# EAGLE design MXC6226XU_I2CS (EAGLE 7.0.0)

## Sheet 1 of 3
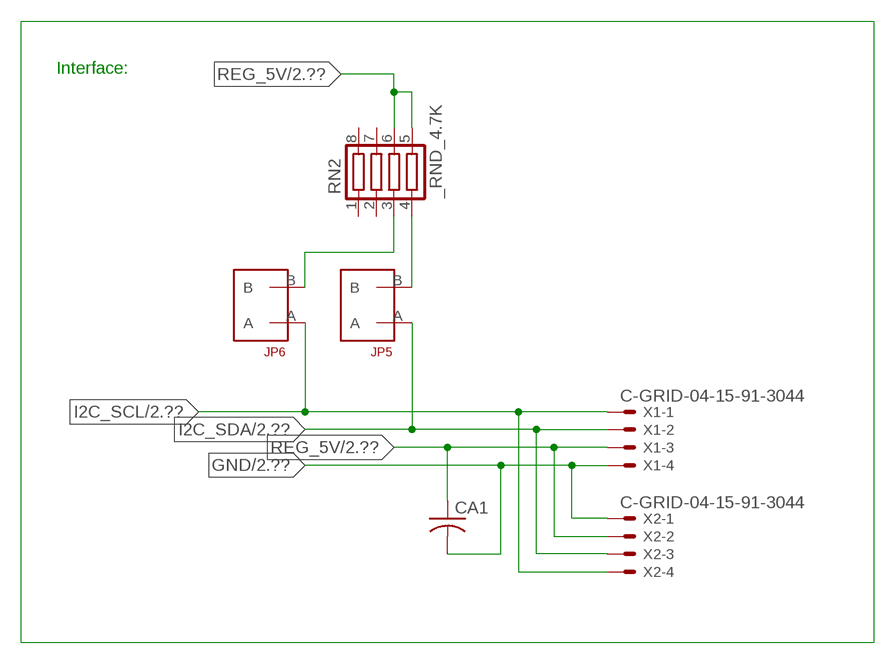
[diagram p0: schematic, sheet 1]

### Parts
CA1  CC1206KRX7R9BB104  [.1UF]
JP5  JUMPER_1X2_2MM  [JUMPER_1X2_2MM]
JP6  JUMPER_1X2_2MM  [JUMPER_1X2_2MM]
RN2  _RND_4.7K  [RND]
X1  C-GRID-04-15-91-3044  [15-91-04]
X2  C-GRID-04-15-91-3044  [15-91-04]

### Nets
GND: CA1.2 X1.4 X2.1 ; also sheet 2,3
I2C_SCL: JP6.A X1.1 X2.4 ; also sheet 2
I2C_SDA: JP5.A X1.2 X2.3 ; also sheet 2
N$1: JP6.B RN2.3
N$2: JP5.B RN2.4
REG_5V: CA1.1 RN2.5 RN2.6 X1.3 X2.2 ; also sheet 2,3
Unconnected: RN2.1 RN2.2 RN2.7 RN2.8

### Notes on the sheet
- Interface:

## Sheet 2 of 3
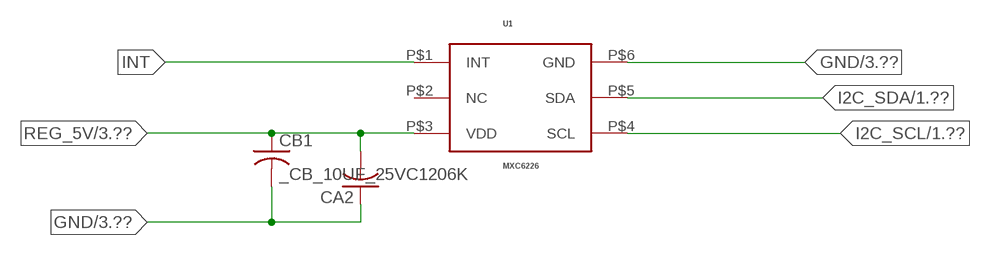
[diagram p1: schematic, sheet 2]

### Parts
CA2  _CA_.10UF_50VC1206K  [_CA_.1UF_50V]
CB1  _CB_10UF_25VC1206K  [_CB_10UF_25V]
U1  MXC6226  [MXC6226]

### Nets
GND: CA2.1 CB1.2 U1.P$6(GND) ; also sheet 1,3
I2C_SCL: U1.P$4(SCL) ; also sheet 1
I2C_SDA: U1.P$5(SDA) ; also sheet 1
INT: U1.P$1(INT)
REG_5V: CA2.2 CB1.1 U1.P$3(VDD) ; also sheet 1,3
Unconnected: U1.P$2(NC)

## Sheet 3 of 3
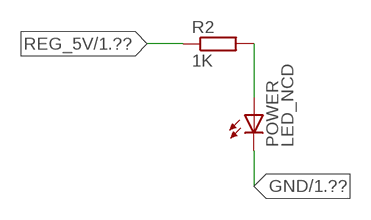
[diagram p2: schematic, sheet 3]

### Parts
POWER  LED_NCD  [CHIPLED_0603]
R2  1K  RESISTOR_SMT-0402  [R402]

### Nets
GND: POWER.C ; also sheet 1,2
N$3: POWER.A R2.2
REG_5V: R2.1 ; also sheet 1,2

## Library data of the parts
CA1 = NCD_ULTIMATE_LIBRARY:CC1206KRX7R9BB104: Capacitor CA .1uF 50V SMT C1206K CC1206KRX7R9BB104
CA2 = NCD_ULTIMATE_LIBRARY:_CA_.10UF_50V: Capacitor .1uF SMT
CB1 = NCD_ULTIMATE_LIBRARY:_CB_10UF_25V: Capacitor 10uF SMT
JP5 JP6 = NCD_ULTIMATE_CONNECTORS:JUMPER_1X2_2MM
POWER = NCD_ULTIMATE_LIBRARY:LED_NCD: LED Digikey 754-1132-2-ND/APT2012SRCPRV
R2 = NCD_ULTIMATE_LIBRARY:RESISTOR_SMT: NCD Resistor
RN2 = NCD_ULTIMATE_LIBRARY:_RND_4.7K: Resistor Array RND SMT 4.7K x 4 Single Resistor Source: http://www.ctscorp.com/components/Datasheets/CTSChipArrayDs.pdf Digikey 742C083472JPTR-ND/742C083472JP; OC_FARNELL: unknown; OC_NEWARK: unknown
U1 = NCD_ULTIMATE_bhaskar:MXC6226: http://www.memsic.com/userfiles/files/Datasheets/Accelerometer-Datasheets/MXC6226XU_Rev_1_3.pdf
X1 X2 = NCD_ULTIMATE_CONNECTORS:C-GRID-04: CONNECTOR 4-Pos I2C wire to board 2.54 mm (0.100") pitch header Digikey WM1342-ND/0015912045; OC_FARNELL: unknown; OC_NEWARK: unknown

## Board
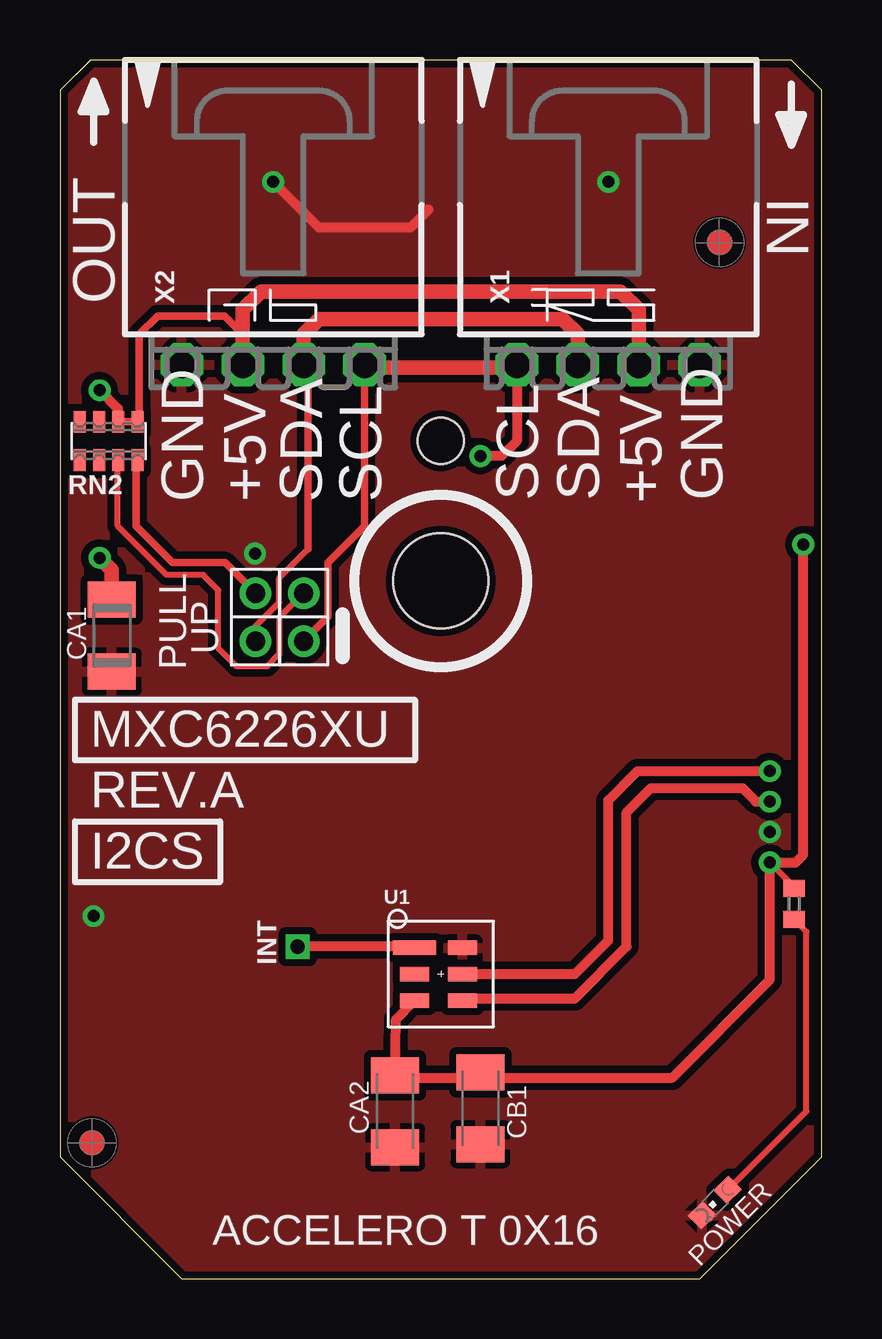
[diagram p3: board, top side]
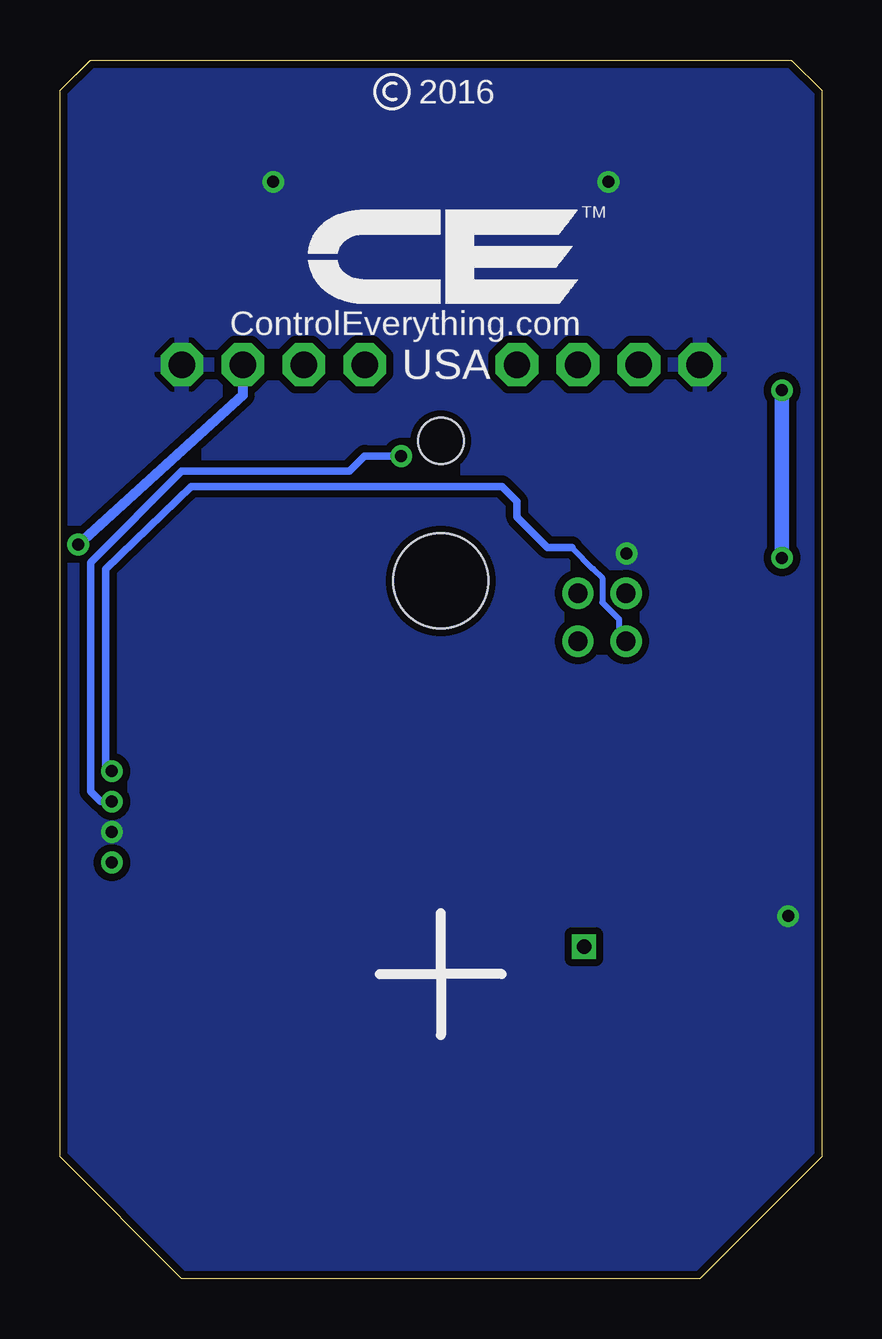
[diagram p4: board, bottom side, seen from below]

Size 31.75 x 50.8 mm. Coordinates in mm from the lower left corner, seen from the top.
Outline: 48 segments
Copper layers (1*16): Top 0.035mm / dielectric 1.5mm / Bottom 0.035mm
Design rules "default": minimum track width 5mil, minimum drill 24mil, track to track 5mil, track to pad 5mil, pad to pad 5mil, via to via 5mil, smd to smd 5mil, copper to edge 10mil, drill to drill 8mil, minimum pad ring 10mil, minimum via ring 8mil, stop-mask expansion 2mil, vias tented up to drill 0mil, thermal gap 10mil
Holes 3.96 mm at 15.88,29.08
Holes 1.91 mm at 15.88,34.92

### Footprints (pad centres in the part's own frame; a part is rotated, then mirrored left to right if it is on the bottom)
.1UF = smd 1.5 x 2: 1 -1.5,0; 2 1.5,0
_CA_.1UF_50V = smd 1.5 x 2: 1 -1.5,0; 2 1.5,0
_CB_10UF_25V = smd 1.5 x 2: 1 -1.5,0; 2 1.5,0
JUMPER_1X2_2MM = drill 0.8: A 0,2; B 0,0
CHIPLED_0603 = smd 0.8 x 0.876: A 0,-0.75; C 0,0.75
R402 = smd 0.7 x 0.9: 1 -0.65,0; 2 0.65,0
RND = smd 0.5 x 0.9: 1 -1.2,-0.8; 2 -0.4,-0.8; 3 0.4,-0.8; 4 1.2,-0.8; 5 1.2,0.8; 6 0.4,0.8; 7 -0.4,0.8; 8 -1.2,0.8
MXC6226 = smd 1.8 x 0.6: P$1 -1.1,1.1 | smd 1.2 x 0.6: P$2 -1.1,0; P$3 -1.1,-1.1; P$4 0.9,-1.1; P$5 0.9,0; P$6 0.9,1.1
15-91-04 = drill 1.1 pad 1.778 octagon: 1 -3.81,-7.62; 2 -1.27,-7.62; 3 1.27,-7.62; 4 3.81,-7.62

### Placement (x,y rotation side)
CA1  2.16,26.81 270 top
CA2  13.97,6.99 90 top
CB1  17.53,7.11 270 top
JP5  8.15,28.58 180 top
JP6  10.16,28.58 180 top
POWER  27.3,3.18 135 top
R2  30.61,15.62 270 top
RN2  2.03,34.92 0 top
U1  15.88,12.7 0 top
U$5  [VISION_REF10]  1.33,5.66 90 top
U$28  [VISION_REF10]  27.5,43.19 90 top
X1  22.86,45.72 0 top
X2  8.89,45.72 0 top

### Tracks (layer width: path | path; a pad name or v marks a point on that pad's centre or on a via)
GND  (via drill 0.5)
  Top 0.406: 15.35,44.57 14.6,43.82 10.8,43.82 v8.89,45.72
  other vias: 22.86,45.72 29.59,18.62 1.4,15.11 8.13,30.23
  pour Top (isolate 0.305): -1.27,0 -1.27,50.8 33.02,50.8 33.02,0
  pour Bottom (isolate 0.305): -5.08,0 -5.08,50.8 35.56,50.8 35.56,0
I2C_SCL  (via drill 0.5)
  Top 0.305: JP6.A 11.18,27.61 11.18,29.85 12.7,31.37 12.7,37.97
  Top 0.406: X2.4 12.7,37.97 | 19.05,37.97 X1.1 19.05,34.93 18.41,34.29 v17.53,34.29 | U1.P$4 16.86,11.68 21.46,11.68 23.62,13.84 23.62,19.43 24.64,20.45 28.45,20.45 29.01,19.89 v29.59,19.89
  Top 0.61: 12.7,37.97 19.05,37.97
  Bottom 0.305: v29.59,19.89 30.05,19.89 30.48,20.32 30.48,29.85 26.67,33.66 19.69,33.66 19.05,34.29 v17.53,34.29
I2C_SDA  (via drill 0.5)
  Top 0.254: JP5.A 8.15,27.2 9.14,28.19 9.14,29.21 10.35,30.42
  Top 0.305: 10.35,30.42 10.35,37.78 X2.3
  Top 0.406: U1.P$5 21.46,12.7 22.86,14.1 22.86,19.94 24.08,21.16 v29.59,21.16
  Top 0.61: X2.3 10.16,39.37 10.8,40.01 20.96,40.01 21.59,39.37 X1.2
  Bottom 0.254: 10.41,30.48 9.52,29.59 9.14,29.21 9.14,28.19 8.45,27.5 8.45,26.87 JP5.A
  Bottom 0.305: 10.41,30.48 11.43,30.48 12.7,31.75 12.7,32.39 13.34,33.02 26.29,33.02 29.85,29.59 29.85,21.41 v29.59,21.16
INT  (via drill 0.6)
  Top 0.406: U1.P$1 14.44,13.84 v9.91,13.84
N$1
  Top 0.254: JP6.B | JP6.B 9.14,27.56 9.14,26.04 8.64,25.53 7.37,25.53 6.6,26.29 6.6,28.7 5.97,29.34 4.45,29.34 2.41,31.37 2.41,34.11 RN2.3
N$2
  Top 0.305: JP5.B 6.88,29.85 4.7,29.85 3.18,31.37 3.18,34.07 RN2.4
N$3
  Top 0.254: POWER.A 31.12,6.99 31.12,14.46 R2.2
REG_5V  (via drill 0.5)
  Top 0.254: v29.59,17.35 30.61,16.33 R2.1
  Top 0.305: 7.62,39.37 7.49,39.37 | RN2.6 RN2.5 3.3,35.8 3.3,39.37 4.06,40.13 6.86,40.13 7.62,39.37 | X2.2 7.62,39.37
  Top 0.406: v1.65,37.03 2.41,36.27 2.41,35.74 RN2.6 | 17.53,8.38 13.95,8.38 CA2.2 14.01,10.81 U1.P$3 | 17.53,8.38 25.53,8.38 29.59,12.45 v29.59,17.35 30.67,17.35 30.99,17.67 v30.99,30.61 | CB1.1 17.4,8.61 17.53,8.38
  Top 0.61: X1.3 24.13,40.39 23.37,41.15 8.38,41.15 7.62,40.39 X2.2 | CA1.1 2.16,29.54 v1.65,30.05
  Bottom 0.406: 24.13,38.23 24.16,38.08 24.13,37.47 24.13,36.83 v30.99,30.61
  Bottom 0.61: v1.65,30.05 v1.65,37.03 | 24.13,38.23 X1.3

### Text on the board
tNames: IN | OUT | GND | +5V | SDA | SCL | SCL | SDA | +5V | GND | UP | PULL | MXC6226XU | REV.A | I2CS | INT | ACCELERO T 0X16
bNames: 2016 | TM | ControlEverything.com | USA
